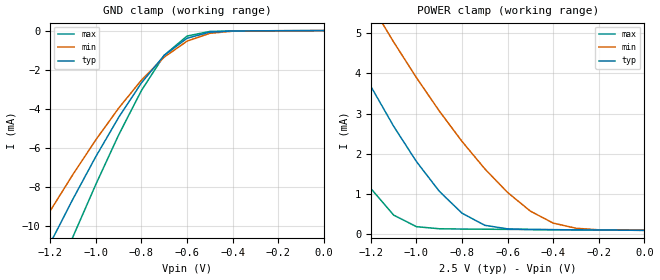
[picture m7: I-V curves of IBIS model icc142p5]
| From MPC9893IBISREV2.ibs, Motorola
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|This model is an Input with a 25,000 ohm Pull_down at 2.5V
[Model]   icc142p5
Model_type   Input
Polarity   Non-Inverting
Vmeas=1.25
Vinl=0.7
Vinh=1.7
| Variable   typ   min   max
C_comp   5p   5p   5p
[Temperature Range]   27.00   100.00   -45.00
[Voltage Range]   2.50V   2.25V   2.75V
[Pulldown Reference]   0.000V   0.000V   0.000V
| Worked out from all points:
|   GND clamp passes 1 mA (typ) near -0.67 V on its own axis
|   POWER clamp passes 1 mA (typ) near -0.89 V on its own axis
[GND_clamp]
|   voltage   I(typ)   I(mim)   I(max)
-2.5V     -43.5mA    -37.6mA    -50mA
-1.3V     -13.21mA   -11.15mA   -16.06mA
-1.2V     -10.86mA   -9.203mA   -13.26mA
-1.1V     -8.591mA   -7.337mA   -10.52mA
-1V       -6.433mA   -5.579mA   -7.854mA
-900mV    -4.435mA   -3.962mA   -5.332mA
-800mV    -2.671mA   -2.531mA   -3.061mA
-700mV    -1.265mA   -1.356mA   -1.26mA
-600mV    -393.2uA   -541.3uA   -279.9uA
-500mV    -78.4uA    -139.9uA   -44.53uA
-400mV    -21.23uA   -31.95uA   -17.01uA
1.08fV    -5.997pA   -194.8pA   -2.759pA
[POWER_clamp]
|   voltage   I(typ)   I(min)   I(max)
-2.5V     21.43mA    20.7mA     21.27mA
-1.6V     8.449mA    9.888mA    6.013mA
-1.5V     7.161mA    8.793mA    4.576mA
-1.3V     4.762mA    6.704mA    2.093mA
-1.2V     3.676mA    5.719mA    1.137mA
-1.1V     2.684mA    4.779mA    476.5uA
-1V       1.807mA    3.893mA    189.9uA
-800mV    523.6uA    2.307mA    130.8uA
-700mV    223.2uA    1.626mA    126.7uA
-500mV    119.8uA    575.5uA    118.8uA
-400mV    114.9uA    278.7uA    114.8uA
1.08fV    99.01uA    99.05uA    99.01uA
